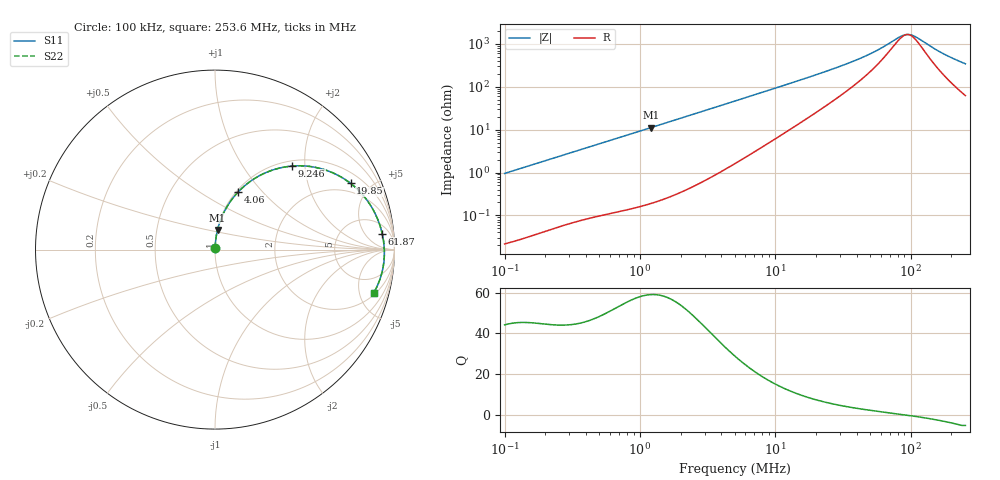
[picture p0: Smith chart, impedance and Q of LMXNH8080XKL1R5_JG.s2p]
! LMXNH8080XKL1R5_JG  S-PARAMETER MODEL  ( General Type )
! Model Generated by TAIYO YUDEN Corporation (https://www.yuden.co.jp/en/)
! Version 1.0
! TAIYO YUDEN Control No. 191025NI43SB-FBB
! Copyright(c) 2019 TAIYO YUDEN CO.,LTD. All Rights Reserved.
! Product Description (link to TY-COMPAS)
! https://ds.yuden.co.jp/TYCOMPAS/or/detail?pn=LMXNH8080XKL1R5NJG&u=M
! Products Name : Inductors
! Characteristics :
!  Inductance : 1.5 uH , SRF(min) : 80 MHz , DC Resistance(max) : 0.0156 Ohm
!  Rated Current : Saturation :6200 mA , Temp Rise : 5300 mA (40 degC)
!  Case Size : 8.0 x 8.0 / 0.315 x 0.315 [mm/inch] , Thickness : 3 / 0.118 [mm/inch]
!  (Conditions: Temperature = 25 degC , DC Bias Current/Voltage = 0A / 0V)
! External Node Assignments :
!  1  o---GGG---o  2
! GND o---------o GND
! Frequency Range : 0.1MHz  -  253.640152MHz  [ 402 STEP ]
# MHz S RI R 50
! Freq[MHz].  S11 Real  S11 Imag  S21 Real  S21 Imag  S12 Real  S12 Imag  S22 Real  S22 Imag
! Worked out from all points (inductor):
!   401 points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, 100 kHz to 253.6 MHz, reference 50 ohm
!   read as one part in series: L = 1.51 uH near 104 kHz
!   highest Q = 59 at 1.205 MHz (marker M1), where L = 1.47 uH
!   self-resonance near 94.28 MHz
!   S11 on the Smith chart (normalised r, x): 100 kHz: 1.00, +0.02; 4.06 MHz: 1.02, +0.75; 9.246 MHz: 1.10, +1.72; 19.85 MHz: 1.50, +3.76; 61.87 MHz: 10, +14; 253.6 MHz: 2.25, -6.78
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0.1  0.000306 0.00952  0.9997 -0.00952  0.9997 -0.00952  0.000306 0.00952
0.371712  0.00198 0.0347  0.998 -0.0347  0.998 -0.0347  0.00198 0.0347
1.20459  0.0141 0.1098  0.9859 -0.1098  0.9859 -0.1098  0.0141 0.1098
1.381698  0.0182 0.1253  0.9818 -0.1253  0.9818 -0.1253  0.0182 0.1253
2.53653  0.0563 0.2203  0.9437 -0.2203  0.9437 -0.2203  0.0563 0.2203
4.059691  0.1308 0.323  0.8692 -0.323  0.8692 -0.323  0.1308 0.323
5.03627  0.187 0.373  0.813 -0.373  0.813 -0.373  0.187 0.373
9.245617  0.4297 0.4655  0.5703 -0.4655  0.5703 -0.4655  0.4297 0.4655
12.90076  0.5866 0.452  0.4134 -0.452  0.4134 -0.452  0.5866 0.452
18.72042  0.7358 0.3833  0.2642 -0.3833  0.2642 -0.3833  0.7358 0.3833
19.85396  0.7551 0.3692  0.2449 -0.3692  0.2449 -0.3692  0.7551 0.3692
27.16539  0.8372 0.288  0.1628 -0.288  0.1628 -0.288  0.8372 0.288
37.90488  0.8915 0.2021  0.1085 -0.2021  0.1085 -0.2021  0.8915 0.2021
48.90263  0.9167 0.1415  0.0833 -0.1415  0.0833 -0.1415  0.9167 0.1415
61.86696  0.9314 0.0893  0.0686 -0.0893  0.0686 -0.0893  0.9314 0.0893
69.58603  0.9364 0.0641  0.0636 -0.0641  0.0636 -0.0641  0.9364 0.0641
88.03362  0.9425 0.0145  0.0575 -0.0145  0.0575 -0.0145  0.9425 0.0145
95.21179  0.9434 -0.00209  0.0566 0.00209  0.0566 0.00209  0.9434 -0.00209
100.977  0.9437 -0.0146  0.0563 0.0146  0.0563 0.0146  0.9437 -0.0146
111.3718  0.9434 -0.0359  0.0566 0.0359  0.0566 0.0359  0.9434 -0.0359
171.3985  0.9281 -0.1361  0.0719 0.1361  0.0719 0.1361  0.9281 -0.1361
253.6402  0.885 -0.24  0.115 0.24  0.115 0.24  0.885 -0.24
